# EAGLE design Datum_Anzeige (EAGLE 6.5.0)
dasdad
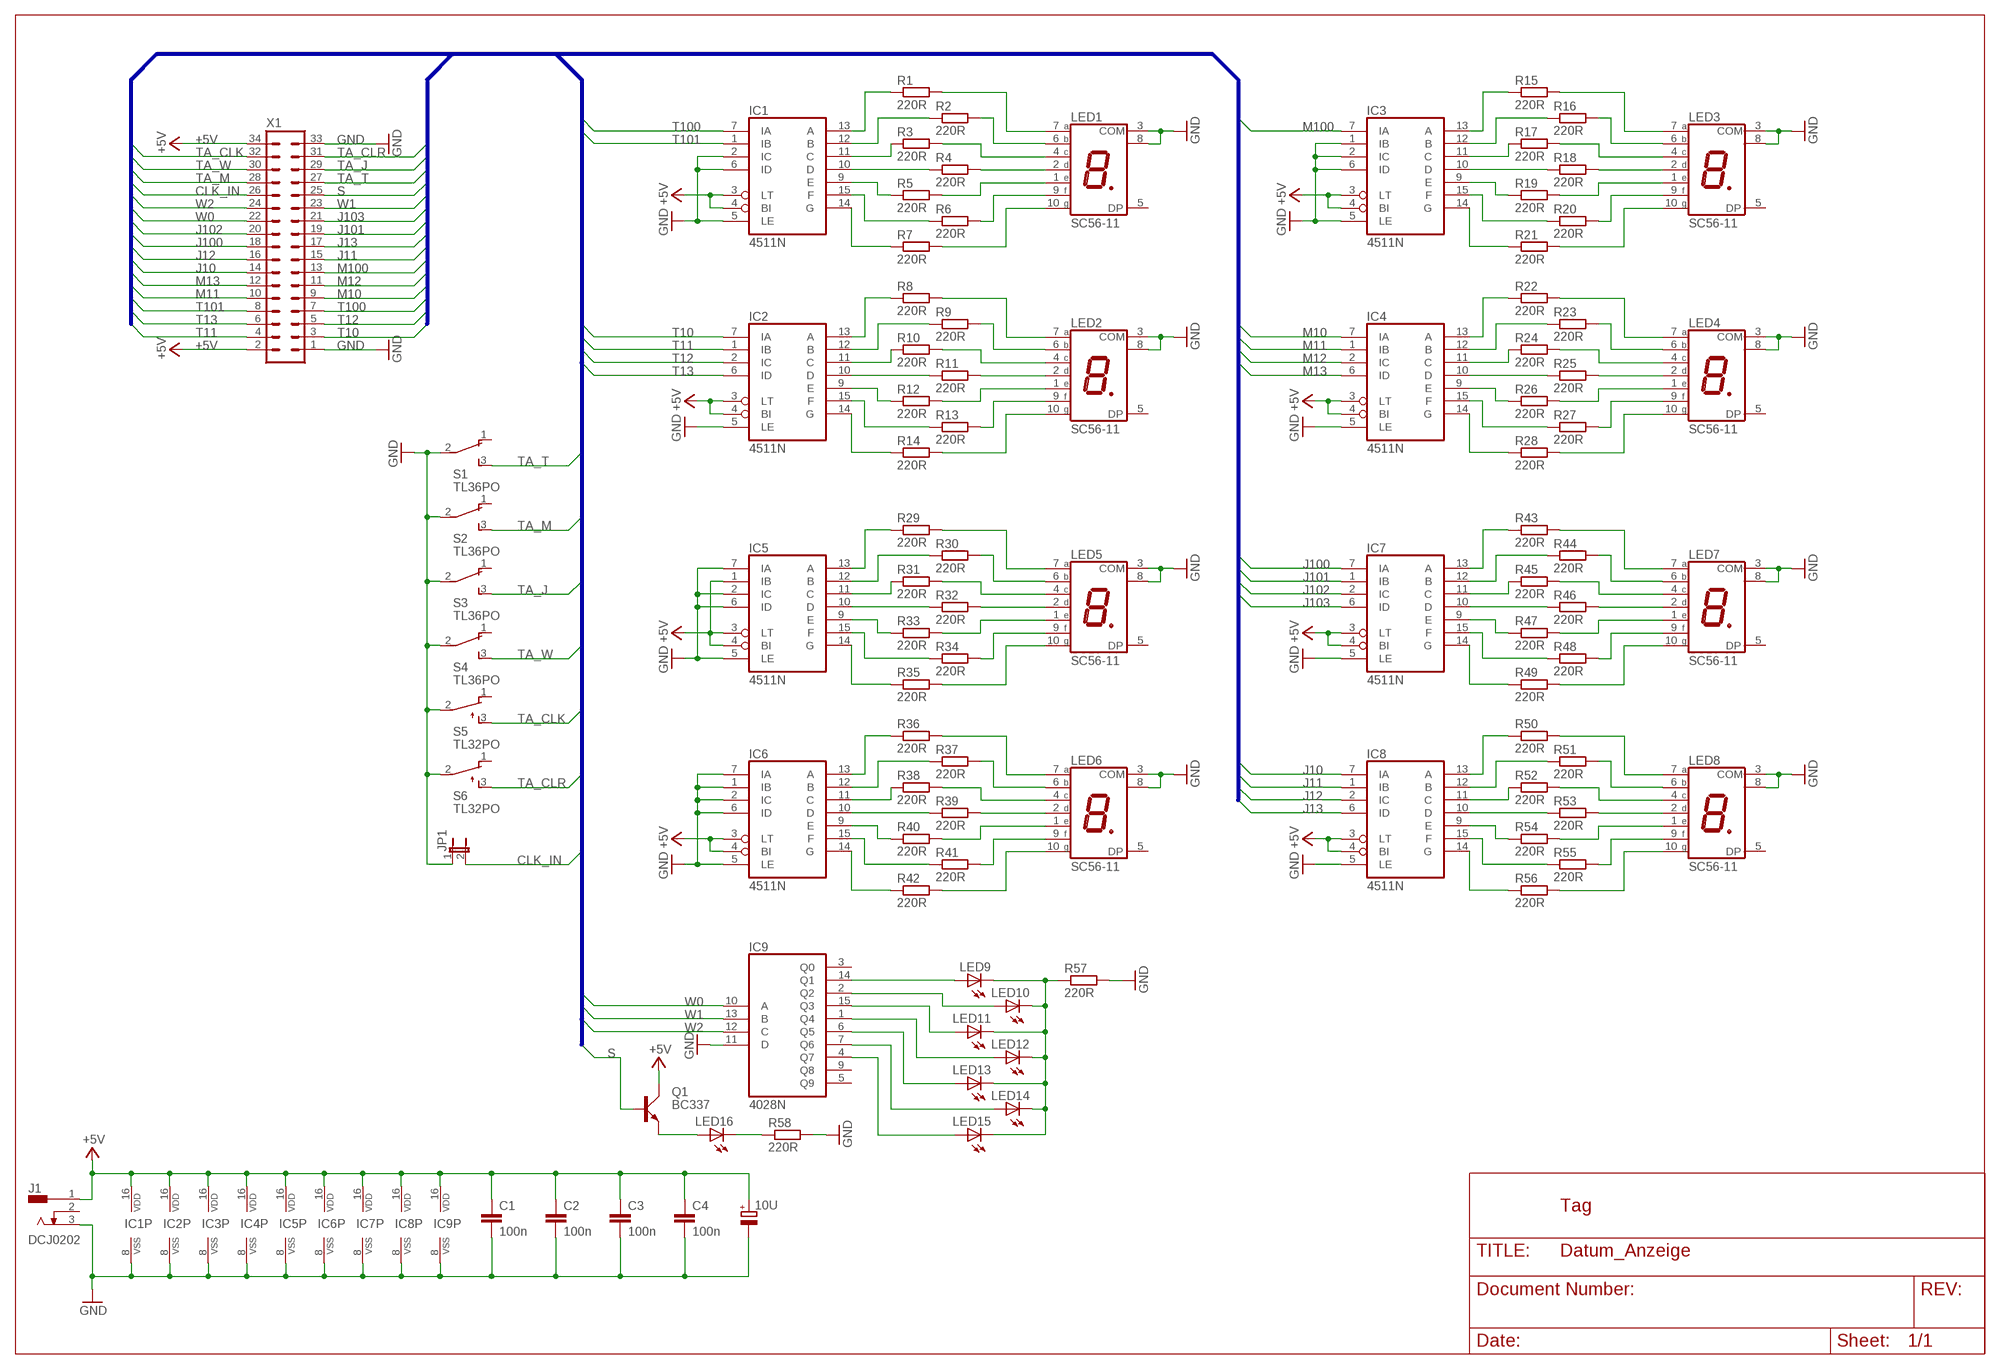
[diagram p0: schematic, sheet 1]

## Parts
10U  CPOL-EUE2.5-7  [E2,5-7]
C1  100n  C-EU025-024X044  [C025-024X044]
C2  100n  C-EU025-024X044  [C025-024X044]
C3  100n  C-EU025-024X044  [C025-024X044]
C4  100n  C-EU025-024X044  [C025-024X044]
IC1  4511N  [DIL16]
IC2  4511N  [DIL16]
IC3  4511N  [DIL16]
IC4  4511N  [DIL16]
IC5  4511N  [DIL16]
IC6  4511N  [DIL16]
IC7  4511N  [DIL16]
IC8  4511N  [DIL16]
IC9  4028N  [DIL16]
J1  DCJ0202  [DCJ0202]
JP1  JP1E  [JP1]
LED1  SC56-11  7-SEG_SA56-11  [SA56-11]
LED2  SC56-11  7-SEG_SA56-11  [SA56-11]
LED3  SC56-11  7-SEG_SA56-11  [SA56-11]
LED4  SC56-11  7-SEG_SA56-11  [SA56-11]
LED5  SC56-11  7-SEG_SA56-11  [SA56-11]
LED6  SC56-11  7-SEG_SA56-11  [SA56-11]
LED7  SC56-11  7-SEG_SA56-11  [SA56-11]
LED8  SC56-11  7-SEG_SA56-11  [SA56-11]
LED9  LED5MM  [LED5MM]
LED10  LED5MM  [LED5MM]
LED11  LED5MM  [LED5MM]
LED12  LED5MM  [LED5MM]
LED13  LED5MM  [LED5MM]
LED14  LED5MM  [LED5MM]
LED15  LED5MM  [LED5MM]
LED16  LED5MM  [LED5MM]
Q1  BC337  [SOT54A]
R1  220R  R-EU_0204/5  [0204/5]
R2  220R  R-EU_0204/5  [0204/5]
R3  220R  R-EU_0204/5  [0204/5]
R4  220R  R-EU_0204/5  [0204/5]
R5  220R  R-EU_0204/5  [0204/5]
R6  220R  R-EU_0204/5  [0204/5]
R7  220R  R-EU_0204/5  [0204/5]
R8  220R  R-EU_0204/5  [0204/5]
R9  220R  R-EU_0204/5  [0204/5]
R10  220R  R-EU_0204/5  [0204/5]
R11  220R  R-EU_0204/5  [0204/5]
R12  220R  R-EU_0204/5  [0204/5]
R13  220R  R-EU_0204/5  [0204/5]
R14  220R  R-EU_0204/5  [0204/5]
R15  220R  R-EU_0204/5  [0204/5]
R16  220R  R-EU_0204/5  [0204/5]
R17  220R  R-EU_0204/5  [0204/5]
R18  220R  R-EU_0204/5  [0204/5]
R19  220R  R-EU_0204/5  [0204/5]
R20  220R  R-EU_0204/5  [0204/5]
R21  220R  R-EU_0204/5  [0204/5]
R22  220R  R-EU_0204/5  [0204/5]
R23  220R  R-EU_0204/5  [0204/5]
R24  220R  R-EU_0204/5  [0204/5]
R25  220R  R-EU_0204/5  [0204/5]
R26  220R  R-EU_0204/5  [0204/5]
R27  220R  R-EU_0204/5  [0204/5]
R28  220R  R-EU_0204/5  [0204/5]
R29  220R  R-EU_0204/5  [0204/5]
R30  220R  R-EU_0204/5  [0204/5]
R31  220R  R-EU_0204/5  [0204/5]
R32  220R  R-EU_0204/5  [0204/5]
R33  220R  R-EU_0204/5  [0204/5]
R34  220R  R-EU_0204/5  [0204/5]
R35  220R  R-EU_0204/5  [0204/5]
R36  220R  R-EU_0204/5  [0204/5]
R37  220R  R-EU_0204/5  [0204/5]
R38  220R  R-EU_0204/5  [0204/5]
R39  220R  R-EU_0204/5  [0204/5]
R40  220R  R-EU_0204/5  [0204/5]
R41  220R  R-EU_0204/5  [0204/5]
R42  220R  R-EU_0204/5  [0204/5]
R43  220R  R-EU_0204/5  [0204/5]
R44  220R  R-EU_0204/5  [0204/5]
R45  220R  R-EU_0204/5  [0204/5]
R46  220R  R-EU_0204/5  [0204/5]
R47  220R  R-EU_0204/5  [0204/5]
R48  220R  R-EU_0204/5  [0204/5]
R49  220R  R-EU_0204/5  [0204/5]
R50  220R  R-EU_0204/5  [0204/5]
R51  220R  R-EU_0204/5  [0204/5]
R52  220R  R-EU_0204/5  [0204/5]
R53  220R  R-EU_0204/5  [0204/5]
R54  220R  R-EU_0204/5  [0204/5]
R55  220R  R-EU_0204/5  [0204/5]
R56  220R  R-EU_0204/5  [0204/5]
R57  220R  R-EU_0204/5  [0204/5]
R58  220R  R-EU_0204/5  [0204/5]
S1  TL36PO  [TL3XPO]
S2  TL36PO  [TL3XPO]
S3  TL36PO  [TL3XPO]
S4  TL36PO  [TL3XPO]
S5  TL32PO  [TL3XPO]
S6  TL32PO  [TL3XPO]
X1  ML34  [ML34]

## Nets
+5V: 10U.+ C1.1 C2.1 C3.1 C4.1 IC1.3(LT) IC1.4(BI) IC1.16(VDD) IC2.3(LT) IC2.4(BI) IC2.16(VDD) IC3.3(LT) IC3.4(BI) IC3.16(VDD) IC4.3(LT) IC4.4(BI) IC4.16(VDD) IC5.1(IB) IC5.3(LT) IC5.4(BI) IC5.16(VDD) IC6.3(LT) IC6.4(BI) IC6.16(VDD) IC7.3(LT) IC7.4(BI) IC7.16(VDD) IC8.3(LT) IC8.4(BI) IC8.16(VDD) IC9.16(VDD) J1.1 Q1.C X1.2 X1.34
CLK_IN: JP1.2 X1.26
GND: 10U.- C1.2 C2.2 C3.2 C4.2 IC1.2(IC) IC1.5(LE) IC1.6(ID) IC1.8(VSS) IC2.5(LE) IC2.8(VSS) IC3.1(IB) IC3.2(IC) IC3.5(LE) IC3.6(ID) IC3.8(VSS) IC4.5(LE) IC4.8(VSS) IC5.2(IC) IC5.5(LE) IC5.6(ID) IC5.7(IA) IC5.8(VSS) IC6.1(IB) IC6.2(IC) IC6.5(LE) IC6.6(ID) IC6.7(IA) IC6.8(VSS) IC7.5(LE) IC7.8(VSS) IC8.5(LE) IC8.8(VSS) IC9.8(VSS) IC9.11(D) J1.3 JP1.1 LED1.3(COM) LED1.8(COM) LED2.3(COM) LED2.8(COM) LED3.3(COM) LED3.8(COM) LED4.3(COM) LED4.8(COM) LED5.3(COM) LED5.8(COM) LED6.3(COM) LED6.8(COM) LED7.3(COM) LED7.8(COM) LED8.3(COM) LED8.8(COM) R57.2 R58.2 S1.2(P) S2.2(P) S3.2(P) S4.2(P) S5.2(P) S6.2(P) X1.1 X1.33
J10: IC8.7(IA) X1.14
J11: IC8.1(IB) X1.15
J12: IC8.2(IC) X1.16
J13: IC8.6(ID) X1.17
J100: IC7.7(IA) X1.18
J101: IC7.1(IB) X1.19
J102: IC7.2(IC) X1.20
J103: IC7.6(ID) X1.21
M10: IC4.7(IA) X1.9
M11: IC4.1(IB) X1.10
M12: IC4.2(IC) X1.11
M13: IC4.6(ID) X1.12
M100: IC3.7(IA) X1.13
N$1: IC1.13(A) R1.1
N$2: LED9.K(C) LED10.K(C) LED11.K(C) LED12.K(C) LED13.K(C) LED14.K(C) LED15.K(C) R57.1
N$3: IC1.12(B) R2.1
N$4: IC1.11(C) R3.1
N$5: IC1.10(D) R4.1
N$6: IC1.9(E) R5.1
N$7: IC1.15(F) R6.1
N$8: IC1.14(G) R7.1
N$9: LED1.2(D) R4.2
N$10: LED1.4(C) R3.2
N$11: LED1.6(B) R2.2
N$12: IC9.2(Q2) LED10.A
N$13: LED1.7(A) R1.2
N$14: LED1.1(E) R5.2
N$15: LED1.9(F) R6.2
N$16: LED1.10(G) R7.2
N$17: IC2.13(A) R8.1
N$18: IC2.12(B) R9.1
N$19: IC2.11(C) R10.1
N$20: IC2.10(D) R11.1
N$21: IC2.9(E) R12.1
N$22: IC2.15(F) R13.1
N$23: IC2.14(G) R14.1
N$24: LED2.2(D) R11.2
N$25: LED2.4(C) R10.2
N$26: LED2.6(B) R9.2
N$27: LED2.7(A) R8.2
N$28: LED2.1(E) R12.2
N$29: LED2.9(F) R13.2
N$30: LED2.10(G) R14.2
N$31: IC9.14(Q1) LED9.A
N$32: IC3.13(A) R15.1
N$33: IC3.12(B) R16.1
N$34: IC3.11(C) R17.1
N$35: IC3.10(D) R18.1
N$36: IC3.9(E) R19.1
N$37: IC3.15(F) R20.1
N$38: IC3.14(G) R21.1
N$39: LED3.2(D) R18.2
N$40: LED3.4(C) R17.2
N$41: LED3.6(B) R16.2
N$42: LED3.7(A) R15.2
N$43: LED3.1(E) R19.2
N$44: LED3.9(F) R20.2
N$45: LED3.10(G) R21.2
N$46: IC4.13(A) R22.1
N$47: IC4.12(B) R23.1
N$48: IC4.11(C) R24.1
N$49: IC4.10(D) R25.1
N$50: IC4.9(E) R26.1
N$51: IC4.15(F) R27.1
N$52: IC4.14(G) R28.1
N$53: LED4.2(D) R25.2
N$54: LED4.4(C) R24.2
N$55: LED4.6(B) R23.2
N$56: LED4.7(A) R22.2
N$57: LED4.1(E) R26.2
N$58: LED4.9(F) R27.2
N$59: LED4.10(G) R28.2
N$60: IC5.13(A) R29.1
N$61: IC5.12(B) R30.1
N$62: IC5.11(C) R31.1
N$63: IC5.10(D) R32.1
N$64: IC5.9(E) R33.1
N$65: IC5.15(F) R34.1
N$66: IC5.14(G) R35.1
N$67: LED5.2(D) R32.2
N$68: LED5.4(C) R31.2
N$69: LED5.6(B) R30.2
N$70: LED5.7(A) R29.2
N$71: LED5.1(E) R33.2
N$72: LED5.9(F) R34.2
N$73: LED5.10(G) R35.2
N$74: IC6.13(A) R36.1
N$75: IC6.12(B) R37.1
N$76: IC6.11(C) R38.1
N$77: IC6.10(D) R39.1
N$78: IC6.9(E) R40.1
N$79: IC6.15(F) R41.1
N$80: IC6.14(G) R42.1
N$81: LED6.2(D) R39.2
N$82: LED6.4(C) R38.2
N$83: LED6.6(B) R37.2
N$84: LED6.7(A) R36.2
N$85: LED6.1(E) R40.2
N$86: LED6.9(F) R41.2
N$87: LED6.10(G) R42.2
N$88: IC7.13(A) R43.1
N$89: IC7.12(B) R44.1
N$90: IC7.11(C) R45.1
N$91: IC7.10(D) R46.1
N$92: IC7.9(E) R47.1
N$93: IC7.15(F) R48.1
N$94: IC7.14(G) R49.1
N$95: LED7.2(D) R46.2
N$96: LED7.4(C) R45.2
N$97: LED7.6(B) R44.2
N$98: LED7.7(A) R43.2
N$99: LED7.1(E) R47.2
N$100: LED7.9(F) R48.2
N$101: LED7.10(G) R49.2
N$102: IC8.13(A) R50.1
N$103: IC8.12(B) R51.1
N$104: IC8.11(C) R52.1
N$105: IC8.10(D) R53.1
N$106: IC8.9(E) R54.1
N$107: IC8.15(F) R55.1
N$108: IC8.14(G) R56.1
N$109: LED8.2(D) R53.2
N$110: LED8.4(C) R52.2
N$111: LED8.6(B) R51.2
N$112: LED8.7(A) R50.2
N$113: LED8.1(E) R54.2
N$114: LED8.9(F) R55.2
N$115: LED8.10(G) R56.2
N$116: IC9.15(Q3) LED11.A
N$117: IC9.1(Q4) LED12.A
N$118: IC9.6(Q5) LED13.A
N$119: IC9.7(Q6) LED14.A
N$120: IC9.4(Q7) LED15.A
N$121: LED16.K(C) R58.1
N$123: LED16.A Q1.E
S: Q1.B X1.25
T10: IC2.7(IA) X1.3
T11: IC2.1(IB) X1.4
T12: IC2.2(IC) X1.5
T13: IC2.6(ID) X1.6
T100: IC1.7(IA) X1.7
T101: IC1.1(IB) X1.8
TA_CLK: S5.3(S) X1.32
TA_CLR: S6.3(S) X1.31
TA_J: S3.3(S) X1.29
TA_M: S2.3(S) X1.28
TA_T: S1.3(S) X1.27
TA_W: S4.3(S) X1.30
W0: IC9.10(A) X1.22
W1: IC9.13(B) X1.23
W2: IC9.12(C) X1.24
Unconnected: IC9.3(Q0) IC9.5(Q9) IC9.9(Q8) J1.2 LED1.5(DP) LED2.5(DP) LED3.5(DP) LED4.5(DP) LED5.5(DP) LED6.5(DP) LED7.5(DP) LED8.5(DP) S1.1(O) S2.1(O) S3.1(O) S4.1(O) S5.1(O) S6.1(O)

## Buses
T10,T11,T12,T13,T100,T101,M100,M10,M11,M12,M13,J100,J101,J102,J103,J10,J11,J12,J13,W0,W1,W2,S,CLK_IN,TA_T,TA_M,TA_J,TA_W,TA_CLK,TA_CLR

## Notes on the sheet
- Tag

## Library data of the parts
10U = rcl:CPOL-EU: POLARIZED CAPACITOR, European symbol
C1-C4 = rcl:C-EU: CAPACITOR, European symbol
IC1-IC8 = 45xx:4511: BCD to 7-segment LATCH/DECODER/DRIVER
IC9 = 40xx:4028: BCD to decimal DECODER
J1 = Brunner:DCJ0202: DC POWER JACK Source: DCJ0202.pdf; OC_FARNELL: unknown; OC_NEWARK: unknown
JP1 = jumper:JP1E: JUMPER
LED1-LED8 = display-kingbright:7-SEG_: Kingbright 14.2mm (0.56 INCH) SINGLE DIGIT NUMERIC DUISPLAY Source: SA56-11EWA(Ver1189471036.pdf; OC_FARNELL: unknown; OC_NEWARK: unknown
LED9-LED16 = led:LED: LED
Q1 = transistor-small-signal:BC337: NPN TRANSISTOR
R1-R58 = rcl:R-EU_: RESISTOR, European symbol
S1-S4 = switch:TL36PO: TINY SWITCH ON - ON Source: http://www2.produktinfo.conrad.com/datenblaetter/700000-724999/705152-da-01-de-Subminiaturschalter_TL_36YO.pdf
S5 S6 = switch:TL32PO: TINY SWITCH ON - MOM Source: http://www2.produktinfo.conrad.com/datenblaetter/700000-724999/705152-da-01-de-Subminiaturschalter_TL_36YO.pdf
X1 = con-harting-ml:ML34: HARTING; OC_FARNELL: unknown; OC_NEWARK: unknown

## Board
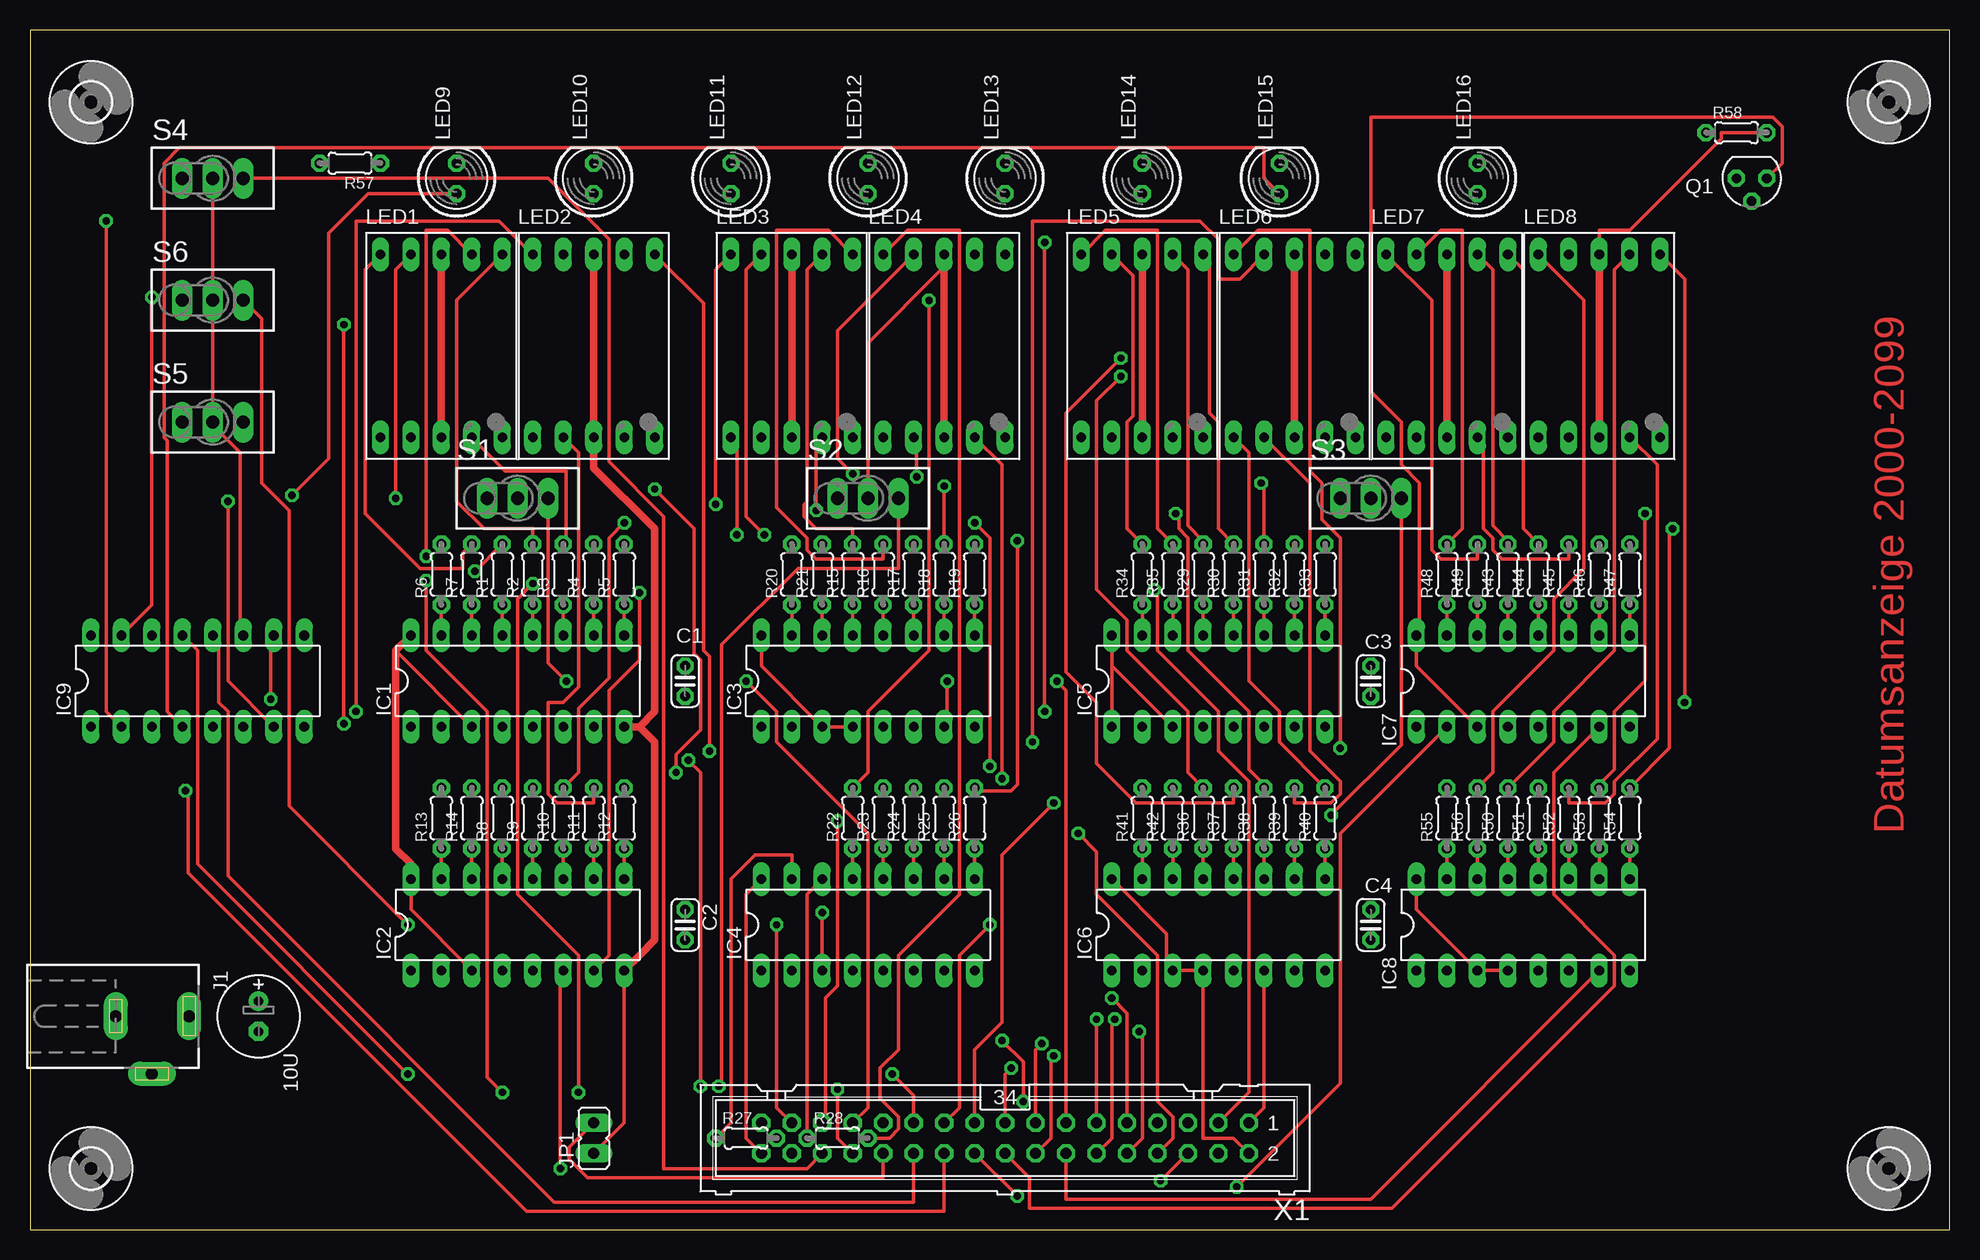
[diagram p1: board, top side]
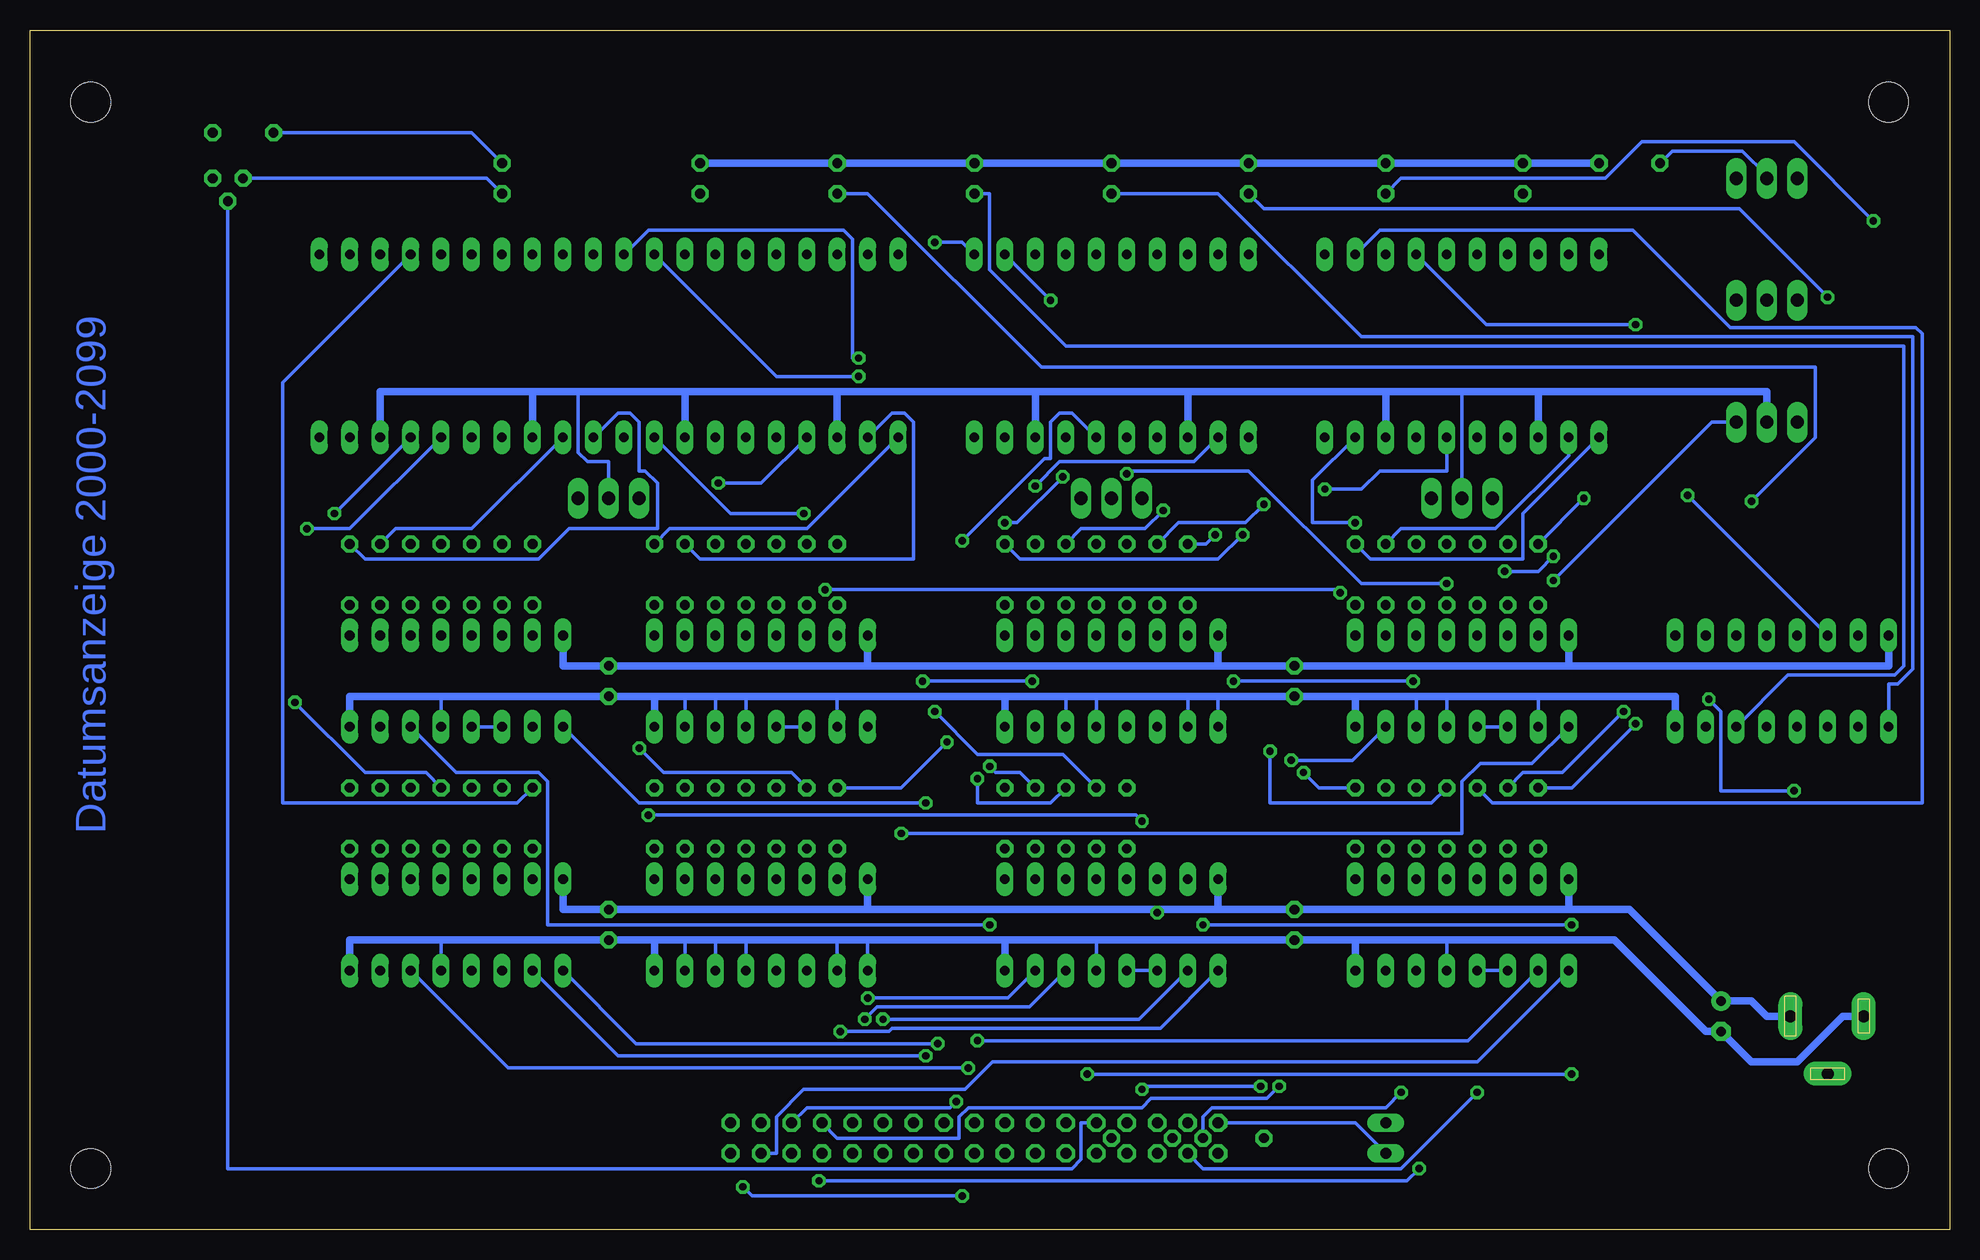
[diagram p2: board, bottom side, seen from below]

Size 160 x 100 mm. Coordinates in mm from the lower left corner, seen from the top.
Outline: 0,0 160,0 160,100 0,100 0,0
Copper layers (1*16): Top 0.035mm / dielectric 1.5mm / Bottom 0.035mm
Design rules "default *": minimum track width 12mil, minimum drill 24mil, track to track 12mil, track to pad 12mil, pad to pad 12mil, via to via 12mil, smd to smd 8mil, copper to edge 40mil, drill to drill 8mil, minimum pad ring 12mil, minimum via ring 10mil, stop-mask expansion 4mil, vias tented up to drill 0mil, thermal gap 10mil

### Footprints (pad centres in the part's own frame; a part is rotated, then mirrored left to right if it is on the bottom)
E2,5-7 = drill 0.813 pad 1.6: + -1.27,0 | drill 0.813 pad 1.6 octagon: - 1.27,0
C025-024X044 = drill 0.813 octagon: 1 -1.27,0; 2 1.27,0
DIL16 = drill 0.813 long: 1 -8.89,-3.81; 2 -6.35,-3.81; 3 -3.81,-3.81; 4 -1.27,-3.81; 5 1.27,-3.81; 6 3.81,-3.81; 7 6.35,-3.81; 8 8.89,-3.81; 9 8.89,3.81; 10 6.35,3.81; 11 3.81,3.81; 12 1.27,3.81; 13 -1.27,3.81; 14 -3.81,3.81; 15 -6.35,3.81; 16 -8.89,3.81
DCJ0202 = drill 1 pad 2 long: 1 0,3.1; 2 4.8,0; 3 0,-3
JP1 = drill 0.914 long: 1 0,-1.27; 2 0,1.27
SA56-11 = drill 0.8 long: 1 -5.08,-7.62; 2 -2.54,-7.62; 3 0,-7.62; 4 2.54,-7.62; 5 5.08,-7.62; 6 5.08,7.62; 7 2.54,7.62; 8 0,7.62; 9 -2.54,7.62; 10 -5.08,7.62
LED5MM = drill 0.813 octagon: A -1.27,0; K 1.27,0
SOT54A = drill 0.813 octagon: B 0,1.905; C -1.27,0; E 1.27,0
0204/5 = drill 0.813 octagon: 1 -2.54,0; 2 2.54,0
TL3XPO = drill 1.1 pad 1.422 long: 1 -2.54,0; 2 0,0; 3 2.54,0
3,3 = hole 3.3: 0,0
ML34 = drill 0.914 octagon: 1 -20.32,-1.27; 2 -20.32,1.27; 3 -17.78,-1.27; 4 -17.78,1.27; 5 -15.24,-1.27; 6 -15.24,1.27; 7 -12.7,-1.27; 8 -12.7,1.27; 9 -10.16,-1.27; 10 -10.16,1.27; 11 -7.62,-1.27; 12 -7.62,1.27; 13 -5.08,-1.27; 14 -5.08,1.27; 15 -2.54,-1.27; 16 -2.54,1.27; 17 0,-1.27; 18 0,1.27; 19 2.54,-1.27; 20 2.54,1.27; 21 5.08,-1.27; 22 5.08,1.27; 23 7.62,-1.27; 24 7.62,1.27; 25 10.16,-1.27; 26 10.16,1.27; 27 12.7,-1.27; 28 12.7,1.27; 29 15.24,-1.27; 30 15.24,1.27; 31 17.78,-1.27; 32 17.78,1.27; 33 20.32,-1.27; 34 20.32,1.27

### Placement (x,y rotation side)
10U  19.05,17.78 270 top
C1  54.61,45.72 270 top
C2  54.61,25.4 270 top
C3  111.76,45.72 270 top
C4  111.76,25.4 270 top
IC1  40.64,45.72 0 top
IC2  40.64,25.4 0 top
IC3  69.85,45.72 0 top
IC4  69.85,25.4 0 top
IC5  99.06,45.72 0 top
IC6  99.06,25.4 0 top
IC7  124.46,45.72 0 top
IC8  124.46,25.4 0 top
IC9  13.97,45.72 0 top
J1  10.16,17.78 270 top
JP1  46.99,7.62 0 top
LED1  34.29,73.66 0 top
LED2  46.99,73.66 0 top
LED3  63.5,73.66 0 top
LED4  76.2,73.66 0 top
LED5  92.71,73.66 0 top
LED6  105.41,73.66 0 top
LED7  118.11,73.66 0 top
LED8  130.81,73.66 0 top
LED9  35.56,87.63 90 top
LED10  46.99,87.63 90 top
LED11  58.42,87.63 90 top
LED12  69.85,87.63 90 top
LED13  81.28,87.63 90 top
LED14  92.71,87.63 90 top
LED15  104.14,87.63 90 top
LED16  120.65,87.63 90 top
Q1  143.51,87.63 180 top
R1  39.37,54.61 90 top
R2  41.91,54.61 90 top
R3  44.45,54.61 90 top
R4  46.99,54.61 90 top
R5  49.53,54.61 90 top
R6  34.29,54.61 90 top
R7  36.83,54.61 90 top
R8  39.37,34.29 90 top
R9  41.91,34.29 90 top
R10  44.45,34.29 90 top
R11  46.99,34.29 90 top
R12  49.53,34.29 90 top
R13  34.29,34.29 90 top
R14  36.83,34.29 90 top
R15  68.58,54.61 90 top
R16  71.12,54.61 90 top
R17  73.66,54.61 90 top
R18  76.2,54.61 90 top
R19  78.74,54.61 90 top
R20  63.5,54.61 90 top
R21  66.04,54.61 90 top
R22  68.58,34.29 90 top
R23  71.12,34.29 90 top
R24  73.66,34.29 90 top
R25  76.2,34.29 90 top
R26  78.74,34.29 90 top
R27  59.69,7.62 0 top
R28  67.31,7.62 0 top
R29  97.79,54.61 90 top
R30  100.33,54.61 90 top
R31  102.87,54.61 90 top
R32  105.41,54.61 90 top
R33  107.95,54.61 90 top
R34  92.71,54.61 90 top
R35  95.25,54.61 90 top
R36  97.79,34.29 90 top
R37  100.33,34.29 90 top
R38  102.87,34.29 90 top
R39  105.41,34.29 90 top
R40  107.95,34.29 90 top
R41  92.71,34.29 90 top
R42  95.25,34.29 90 top
R43  123.19,54.61 90 top
R44  125.73,54.61 90 top
R45  128.27,54.61 90 top
R46  130.81,54.61 90 top
R47  133.35,54.61 90 top
R48  118.11,54.61 90 top
R49  120.65,54.61 90 top
R50  123.19,34.29 90 top
R51  125.73,34.29 90 top
R52  128.27,34.29 90 top
R53  130.81,34.29 90 top
R54  133.35,34.29 90 top
R55  118.11,34.29 90 top
R56  120.65,34.29 90 top
R57  26.67,88.9 180 top
R58  142.24,91.44 0 top
S1  40.64,60.96 0 top
S2  69.85,60.96 0 top
S3  111.76,60.96 0 top
S4  15.24,87.63 0 top
S5  15.24,67.31 0 top
S6  15.24,77.47 0 top
U$1  [3,3]  5.08,93.98 0 top
U$2  [3,3]  5.08,5.08 0 top
U$3  [3,3]  154.94,93.98 0 top
U$4  [3,3]  154.94,5.08 0 top
U$5  [A4L-LOC]  not placed on the board
X1  81.28,7.62 180 top

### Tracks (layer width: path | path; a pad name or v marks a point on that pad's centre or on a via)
+5V  (via drill 0.61)
  Top 0.305: X1.2 100.33,7.62 97.79,7.62 IC6.4 IC6.3 94.74,22.1 94.74,24.64 IC6.16 | IC8.4 IC8.3 115.57,26.67 IC8.16 | IC3.4 IC3.3 60.96,46.99 IC3.16 | IC5.16 90.17,46.99 | 90.17,46.99 IC5.1 | Q1.C 146.05,88.9 146.05,91.95 145.29,92.71 111.76,92.71 111.76,69.85 114.3,67.31 114.3,63.75 115.82,62.23 115.82,49.78 IC7.16 115.57,46.99 IC7.3 | X1.34 59.69,7.62 59.69,27.94 IC4.16 | IC2.3 31.75,26.67 31.75,28.96 IC2.16 | IC1.3 30.73,48.01 30.48,48.01 | v66.04,26.42 IC4.3 | 90.17,46.99 IC5.3
  Top 0.61: IC2.16 31.75,30.48 30.48,31.75 30.48,48.01 30.48,48.26 IC1.16
  Bottom 0.305: IC7.4 IC7.3 | IC5.4 IC5.3 | IC4.4 IC4.3 | IC1.4 IC1.3 | IC2.4 IC2.3 | v66.04,26.42 66.04,26.67
  Bottom 0.61: IC9.16 5.08,46.99 31.75,46.99 | 31.75,46.99 C1.1 60.96,46.99 | 60.96,46.99 90.17,46.99 | 90.17,46.99 C3.1 115.57,46.99 IC7.16 | IC5.16 90.17,46.99 | IC3.16 60.96,48.26 60.96,46.99 | IC1.16 31.75,46.99 | IC2.16 31.75,26.67 | 31.75,26.67 C2.1 60.96,26.67 | 60.96,26.67 66.04,26.67 90.17,26.67 | 90.17,26.67 C4.1 115.57,26.67 IC8.16 | IC6.16 90.17,26.67 | IC4.16 60.96,26.67 | 31.75,26.67 26.67,26.67 10U.+ 16.51,19.05 15.24,17.78 J1.1
CLK_IN
  Top 0.305: JP1.2 44.96,6.86 44.96,5.84 46.48,4.32 71.12,4.32 X1.26
GND
  Top 0.305: S4.2 S6.2 S5.2 15.24,67.06 17.53,64.77 17.53,49.78 IC9.11 | R58.2 140.97,91.44 140.97,90.93 133.35,83.31 130.81,83.31 130.81,81.53 LED8.8 | X1.1 102.87,10.16 IC6.6 | S2.2 69.85,73.91 75.95,80.01 LED4.8 | JP1.1 49.53,8.89 49.53,21.34 IC2.8
  Top 0.61: IC2.8 50.8,22.86 52.07,24.13 52.07,40.64 50.8,41.91 | 50.8,41.91 IC1.8 50.8,41.91 | LED1.8 LED1.3 | LED2.8 LED2.3 46.99,63.5 52.07,58.42 52.07,43.18 50.8,41.91 | LED3.8 LED3.3 | LED4.8 LED4.3 | LED5.8 LED5.3 | LED6.8 LED6.3 | LED7.8 LED7.3 | LED8.8 LED8.3
  Bottom 0.305: R57.2 23.11,89.92 17.27,89.92 15.24,87.88 S4.2 | JP1.1 49.53,8.89 X1.33 | IC2.5 41.91,23.88 41.91,24.13 | IC1.2 34.29,44.2 34.29,44.45 | IC1.5 41.91,44.2 41.91,44.45 | IC1.6 44.45,44.2 44.45,44.45 | IC4.5 71.12,23.88 71.12,24.13 | IC3.1 60.96,44.2 60.96,44.45 | IC3.2 63.5,44.2 63.5,44.45 | IC3.5 71.12,44.2 71.12,44.45 | IC3.6 73.66,44.2 73.66,44.45 | IC6.1 90.17,23.88 90.17,24.13 | IC6.2 92.71,23.88 92.71,24.13 | IC5.2 92.71,44.2 92.71,44.45 | IC6.5 100.33,23.88 100.33,24.13 | IC6.6 102.87,23.88 102.87,24.13 | IC6.7 105.41,23.88 105.41,24.13 | IC8.5 125.73,23.88 125.73,24.13 | IC5.5 100.33,44.2 100.33,44.45 | IC5.6 102.87,44.2 102.87,44.45 | IC5.7 105.41,44.2 105.41,44.45 | IC7.5 125.73,44.2 125.73,44.45 | S1.2 40.64,69.6 40.64,69.85 | S3.2 111.76,64.01 113.54,64.01 114.3,64.77 114.3,69.6 114.3,69.85
  Bottom 0.61: IC9.8 22.86,44.45 34.29,44.45 41.91,44.45 44.45,44.45 49.53,44.45 | 49.53,44.45 C1.2 60.96,44.45 63.5,44.45 71.12,44.45 73.66,44.45 78.74,44.45 | 78.74,44.45 92.71,44.45 100.33,44.45 102.87,44.45 105.41,44.45 107.95,44.45 | 107.95,44.45 C3.2 125.73,44.45 133.35,44.45 IC7.8 | IC5.8 107.95,44.45 | IC3.8 78.74,44.45 | IC1.8 49.53,44.45 | IC2.8 49.53,24.13 | 49.53,24.13 C2.2 71.12,24.13 78.74,24.13 | 78.74,24.13 90.17,24.13 92.71,24.13 100.33,24.13 102.87,24.13 105.41,24.13 107.95,24.13 | 107.95,24.13 C4.2 125.73,24.13 133.35,24.13 IC8.8 | IC6.8 107.95,24.13 | IC4.8 78.74,24.13 | 49.53,24.13 41.91,24.13 27.94,24.13 20.32,16.51 10U.- 17.78,15.24 16.51,13.97 12.7,13.97 8.89,17.78 7.62,17.78 J1.3 | S5.2 15.24,69.85 34.29,69.85 | 34.29,69.85 40.64,69.85 46.99,69.85 | 46.99,69.85 63.5,69.85 | 63.5,69.85 76.2,69.85 | 76.2,69.85 92.71,69.85 | 92.71,69.85 105.41,69.85 | 105.41,69.85 114.3,69.85 118.11,69.85 | 118.11,69.85 130.81,69.85 LED8.3 | LED7.3 118.11,69.85 | LED6.3 105.41,69.85 | LED5.3 92.71,69.85 | LED4.3 76.2,69.85 | LED3.3 63.5,69.85 | LED2.3 46.99,69.85 | LED1.3 34.29,69.85
J10
  Top 0.305: IC8.7 111.76,2.54 86.36,2.54 X1.14
J11  (via drill 0.61)
  Top 0.305: v84.33,15.49 83.82,14.99 X1.15
  Bottom 0.305: IC8.1 109.47,15.49 v84.33,15.49
J12  (via drill 0.61)
  Top 0.305: v85.34,14.48 85.09,14.22 85.09,7.62 X1.16
  Bottom 0.305: IC8.2 111,14.48 v85.34,14.48
J13  (via drill 0.61)
  Top 0.305: v81.79,13.46 81.28,12.95 X1.17
  Bottom 0.305: IC8.6 120.14,13.46 v81.79,13.46
J100
  Top 0.305: IC7.7 127,38.1 127,27.94 132.08,22.86 132.08,20.32 113.54,1.78 83.31,1.78 83.31,4.32 X1.18
J101  (via drill 0.61)
  Top 0.305: v85.34,35.56 81.03,31.24 81.03,17.27 78.74,14.99 X1.19
  Bottom 0.305: IC7.1 109.22,35.56 v85.34,35.56
J102  (via drill 0.61)
  Top 0.305: IC7.2 109.22,33.02 109.22,12.19 v100.58,3.56 | X1.20 v82.3,2.79
  Bottom 0.305: v100.58,3.56 99.82,2.79 v82.3,2.79
J103  (via drill 0.61)
  Top 0.305: v80.01,25.4 77.47,22.86 77.47,10.16 X1.21
  Bottom 0.305: IC7.6 124.46,38.1 117.6,38.1 116.84,37.34 116.84,25.4 v80.01,25.4
M10  (via drill 0.61)
  Top 0.305: v90.17,19.3 91.44,18.03 X1.9
  Bottom 0.305: IC4.7 78.49,19.3 v90.17,19.3
M11  (via drill 0.61)
  Top 0.305: v92.46,16.51 92.71,16.26 92.71,7.62 X1.10
  Bottom 0.305: IC4.1 65.79,16.76 88.14,16.76 88.39,16.51 v92.46,16.51
M12  (via drill 0.61)
  Top 0.305: X1.11 v88.9,17.53
  Bottom 0.305: IC4.2 67.56,17.53 v88.9,17.53
M13  (via drill 0.61)
  Top 0.305: v90.42,17.53 90.17,17.27 90.17,7.62 X1.12
  Bottom 0.305: IC4.6 76.71,18.54 89.41,18.54 v90.42,17.53
M100  (via drill 0.61)
  Top 0.305: IC3.7 76.45,42.16 v76.45,45.72 | v85.6,45.72 86.36,44.96 X1.13
  Bottom 0.305: v85.6,45.72 v76.45,45.72
N$1
  Top 0.305: R1.1 IC1.13
N$2
  Bottom 0.61: LED15.K LED14.K LED13.K LED12.K LED11.K LED10.K LED9.K R57.1
N$3
  Top 0.305: R2.1 IC1.12
N$4
  Top 0.305: R3.1 IC1.11
N$5
  Top 0.305: R4.1 IC1.10
N$6
  Top 0.305: R5.1 IC1.9
N$7
  Top 0.305: R6.1 IC1.15
N$8
  Top 0.305: R7.1 IC1.14
N$9
  Bottom 0.305: LED1.2 31.75,64.52 37.85,58.42 45.72,58.42 R4.2
N$10
  Top 0.305: LED1.4 39.62,63.25 44.7,63.25 44.7,57.4 R3.2
N$11
  Top 0.305: LED1.6 35.56,77.47 35.56,60.71 37.85,58.42 41.91,58.42 R2.2
N$12  (via drill 0.61)
  Top 0.305: IC9.2 6.35,43.18 v6.35,84.07
  Bottom 0.305: v6.35,84.07 12.95,90.68 25.65,90.68 28.7,87.63 45.72,87.63 LED10.A
N$13  (via drill 0.61)
  Top 0.305: LED1.7 34.8,83.31 33.02,83.31 v33.02,56.13 | R1.2 v37.08,54.86
  Bottom 0.305: v33.02,56.13 34.29,54.86 v37.08,54.86
N$14
  Bottom 0.305: LED1.1 35.56,59.69 35.56,55.88 48.26,55.88 R5.2
N$15  (via drill 0.61)
  Top 0.305: LED1.9 30.48,80.01 v30.48,60.96
  Bottom 0.305: R6.2 v30.48,60.96
N$16
  Top 0.305: LED1.10 27.94,80.01 27.94,59.69 32.51,55.12 36.07,55.12 36.07,56.39 R7.2
N$17
  Top 0.305: R8.1 IC2.13
N$18
  Top 0.305: R9.1 IC2.12
N$19
  Top 0.305: R10.1 IC2.11
N$20
  Top 0.305: R11.1 IC2.10
N$21
  Top 0.305: R12.1 IC2.9
N$22
  Top 0.305: R13.1 IC2.15
N$23
  Top 0.305: R14.1 IC2.14
N$24
  Top 0.305: LED2.2 45.72,64.77 45.72,45.21 44.45,43.94 43.18,43.94 43.18,36.32 43.94,35.56 46.99,35.56 R11.2
N$25  (via drill 0.61)
  Top 0.305: v49.53,58.93 48.26,57.66 48.26,45.97 45.72,43.43 45.72,38.1 R10.2
  Bottom 0.305: LED2.4 53.09,62.48 53.09,58.93 v49.53,58.93
N$26  (via drill 0.61)
  Top 0.305: LED2.6 56.13,77.22 56.13,48.26 56.64,47.75 v56.64,39.88
  Bottom 0.305: v56.64,39.88 56.64,35.56 43.18,35.56 R9.2
N$27
  Bottom 0.305: LED2.7 47.5,83.31 26.42,83.31 18.29,75.18 2.79,75.18 2.29,74.68 2.29,35.56 38.1,35.56 R8.2
N$28  (via drill 0.61)
  Top 0.305: v52.07,61.72 55.37,58.42 55.37,48.01 55.88,47.5 55.88,41.66 53.85,39.62 v53.85,38.1
  Bottom 0.305: LED2.1 41.91,63.25 47.5,63.25 49.02,61.72 v52.07,61.72 | v53.85,38.1 52.58,36.83 R12.2
N$29  (via drill 0.61)
  Top 0.305: v26.16,42.16 v26.16,75.44
  Bottom 0.305: LED2.9 38.61,75.44 v26.16,75.44 | v26.16,42.16 31.5,36.83 R13.2
N$30  (via drill 0.61)
  Top 0.305: LED2.10 39.12,84.07 27.18,84.07 v27.18,43.18
  Bottom 0.305: v27.18,43.18 32.26,38.1 35.56,38.1 R14.2
N$31  (via drill 0.61)
  Top 0.305: v21.84,61.21 24.89,64.26 24.89,83.06 28.19,86.36 LED9.A
  Bottom 0.305: v21.84,61.21 IC9.14
N$32
  Top 0.305: R15.1 IC3.13
N$33
  Top 0.305: R16.1 IC3.12
N$34
  Top 0.305: R17.1 IC3.11
N$35
  Top 0.305: R18.1 IC3.10
N$36
  Top 0.305: R19.1 IC3.9
N$37
  Top 0.305: R20.1 IC3.15
N$38
  Top 0.305: R21.1 IC3.14
N$39  (via drill 0.61)
  Top 0.305: R18.2 v76.2,61.98
  Bottom 0.305: LED3.2 62.99,64.01 74.17,64.01 v76.2,61.98
N$40  (via drill 0.61)
  Top 0.305: LED3.4 65.53,65.53 v65.53,59.94
  Bottom 0.305: v65.53,59.94 67.06,58.42 72.39,58.42 R17.2
N$41
  Top 0.305: LED3.6 66.55,83.31 62.23,83.31 62.23,60.2 64.77,57.66 64.77,56.64 65.53,55.88 71.12,55.88 R16.2
N$42
  Top 0.305: LED3.7 64.77,80.01 64.77,60.71 64.52,60.45 64.52,59.44 65.53,58.42 68.58,58.42 R15.2
N$43  (via drill 0.61)
  Top 0.305: LED3.1 58.93,65.53 v58.93,57.91
  Bottom 0.305: v58.93,57.91 60.96,55.88 77.47,55.88 R19.2
N$44  (via drill 0.61)
  Top 0.305: LED3.9 59.69,80.01 59.69,59.44 v61.21,57.91
  Bottom 0.305: v61.21,57.91 61.98,57.15 R20.2
N$45  (via drill 0.61)
  Top 0.305: LED3.10 57.15,80.01 v57.15,60.45
  Bottom 0.305: v57.15,60.45 58.67,58.93 64.26,58.93 R21.2
N$46
  Top 0.305: R22.1 IC4.13
N$47
  Top 0.305: R23.1 IC4.12
N$48
  Top 0.305: R24.1 IC4.11
N$49
  Top 0.305: R25.1 IC4.10
N$50
  Top 0.305: R26.1 IC4.9
N$51
  Top 0.305: R27.1 58.42,8.89 58.42,29.21 60.45,31.24 63.5,31.24 IC4.15
N$52
  Top 0.305: R28.1 64.77,27.94 IC4.14
N$53  (via drill 0.61)
  Top 0.305: LED4.2 73.91,65.79 v73.91,62.74 | v78.74,58.93 80.01,57.66 v80.01,38.61
  Bottom 0.305: v73.91,62.74 77.72,58.93 v78.74,58.93 | v80.01,38.61 79.5,38.1 77.47,38.1 R25.2
N$54  (via drill 0.61)
  Top 0.305: LED4.4 81.03,63.75 v81.03,37.59
  Bottom 0.305: v81.03,37.59 81.03,35.56 74.93,35.56 R24.2
N$55  (via drill 0.61)
  Top 0.305: v84.58,43.18 v84.58,82.3
  Bottom 0.305: LED4.6 82.3,82.3 v84.58,82.3 | v84.58,43.18 81.03,39.62 73.91,39.62 R23.2
N$56  (via drill 0.61)
  Top 0.305: v74.93,77.47 74.93,48.26 69.85,43.18 69.85,38.1 R22.2
  Bottom 0.305: v74.93,77.47 LED4.7
N$57  (via drill 0.61)
  Top 0.305: v82.3,57.4 82.3,37.08 81.79,36.58 78.74,36.58 R26.2
  Bottom 0.305: LED4.1 73.15,68.07 74.17,68.07 74.93,67.31 74.93,64.26 75.44,64.26 v82.3,57.4
N$58  (via drill 0.61)
  Top 0.305: LED4.9 67.31,74.93 67.31,64.26 v68.58,62.99 | v41.91,53.85 40.64,52.58 40.64,27.94 45.72,22.86 v45.72,11.43
  Bottom 0.305: v68.58,62.99 68.33,63.25 58.42,63.25 49.02,53.85 v41.91,53.85 | v45.72,11.43 46.99,10.16 61.47,10.16 62.23,9.4 R27.2
N$59
  Top 0.305: LED4.10 73.15,83.31 77.47,83.31 77.47,27.94 72.39,22.86 72.39,14.99 70.87,13.46 70.87,10.92 72.39,9.4 72.39,8.38 71.63,7.62 R28.2
N$60
  Top 0.305: R29.1 IC5.13
N$61
  Top 0.305: R30.1 IC5.12
N$62
  Top 0.305: R31.1 IC5.11
N$63
  Top 0.305: R32.1 IC5.10
N$64
  Top 0.305: R33.1 IC5.9
N$65
  Top 0.305: R34.1 IC5.15
N$66
  Top 0.305: R35.1 IC5.14
N$67
  Bottom 0.305: LED5.2 88.14,68.07 87.12,68.07 86.36,67.31 86.36,55.88 104.14,55.88 R32.2
N$68  (via drill 0.61)
  Top 0.305: v102.62,62.23 102.87,61.98 R31.2
  Bottom 0.305: LED5.4 99.06,62.23 v102.62,62.23
N$69
  Top 0.305: LED5.6 98.3,80.77 98.3,68.07 99.06,67.31 99.06,58.42 R30.2
N$70
  Top 0.305: LED5.7 96.52,80.01 96.52,58.67 97.79,57.4 R29.2
N$71
  Bottom 0.305: LED5.1 95.25,58.42 106.68,58.42 R33.2
N$72
  Top 0.305: LED5.9 91.95,79.5 91.95,67.82 91.44,67.31 91.44,58.42 R34.2
N$73
  Top 0.305: LED5.10 89.66,83.31 93.98,83.31 93.98,58.42 R35.2
N$74
  Top 0.305: R36.1 IC6.13
N$75
  Top 0.305: R37.1 IC6.12
N$76
  Top 0.305: R38.1 IC6.11
N$77
  Top 0.305: R39.1 IC6.10
N$78
  Top 0.305: R40.1 IC6.9
N$79
  Top 0.305: R41.1 IC6.15
N$80
  Top 0.305: R42.1 IC6.14
N$81
  Top 0.305: LED6.2 106.68,62.23 106.68,39.88 109.22,37.34 109.22,36.32 108.46,35.56 105.41,35.56 R39.2
N$82  (via drill 0.61)
  Top 0.305: v95.5,59.69 95.76,59.44 95.76,58.42 96.52,57.66 96.52,48.26 101.6,43.18 101.6,38.35 102.87,37.08 R38.2
  Bottom 0.305: LED6.4 101.6,59.69 v95.5,59.69
N$83  (via drill 0.61)
  Top 0.305: v90.93,72.64 86.36,68.07 86.36,46.48 88.9,43.94 88.9,38.86 92.2,35.56 100.33,35.56 R37.2
  Bottom 0.305: LED6.6 108.46,83.31 92.2,83.31 91.44,82.55 91.44,72.64 v90.93,72.64
N$84  (via drill 0.61)
  Top 0.305: v90.93,71.12 88.9,69.09 88.9,53.34 91.44,50.8 91.44,48.26 96.52,43.18 96.52,38.1 R36.2
  Bottom 0.305: LED6.7 97.79,71.12 v90.93,71.12
N$85
  Top 0.305: LED6.1 101.6,64.77 101.6,45.72 104.14,43.18 104.14,40.64 R40.2
N$86  (via drill 0.61)
  Top 0.305: LED6.9 100.84,79.25 99.06,79.25 99.06,82.55 97.54,84.07 83.57,84.07 v83.57,40.64
  Bottom 0.305: v83.57,40.64 87.38,36.83 R41.2
N$87  (via drill 0.61)
  Top 0.305: LED6.10 102.36,83.31 106.68,83.31 106.68,63.25 107.7,62.23 107.7,59.18 109.22,57.66 v109.22,40.13
  Bottom 0.305: v109.22,40.13 107.19,38.1 96.52,38.1 R42.2
N$88
  Top 0.305: R43.1 IC7.13
N$89
  Top 0.305: R44.1 IC7.12
N$90
  Top 0.305: R45.1 IC7.11
N$91
  Top 0.305: R46.1 IC7.10
N$92
  Top 0.305: R47.1 IC7.9
N$93
  Top 0.305: R48.1 IC7.15
N$94
  Top 0.305: R49.1 IC7.14
N$95
  Bottom 0.305: LED7.2 123.19,58.42 129.54,58.42 R46.2
N$96
  Top 0.305: LED7.4 121.16,65.53 121.16,58.42 121.92,57.66 121.92,56.64 122.68,55.88 128.27,55.88 R45.2
N$97
  Top 0.305: LED7.6 124.46,80.01 124.46,58.42 R44.2
N$98
  Top 0.305: LED7.7 121.92,80.01 121.92,58.67 123.19,57.4 R43.2
N$99
  Bottom 0.305: LED7.1 111,68.07 109.98,68.07 109.22,67.31 109.22,63.25 108.71,63.25 107.7,62.23 107.7,58.42 115.06,58.42 117.6,55.88 132.08,55.88 R47.2
N$100
  Top 0.305: LED7.9 117.6,83.31 119.38,83.31 119.38,58.42 R48.2
N$101
  Top 0.305: LED7.10 116.84,77.47 116.84,56.64 117.6,55.88 120.65,55.88 R49.2
N$102
  Top 0.305: R50.1 IC8.13
N$103
  Top 0.305: R51.1 IC8.12
N$104
  Top 0.305: R52.1 IC8.11
N$105
  Top 0.305: R53.1 IC8.10
N$106
  Top 0.305: R54.1 IC8.9
N$107
  Top 0.305: R55.1 IC8.15
N$108
  Top 0.305: R56.1 IC8.14
N$109  (via drill 0.61)
  Top 0.305: v134.62,59.69 134.62,45.72 132.08,43.18 132.08,38.35 130.81,37.08 R53.2
  Bottom 0.305: v134.62,59.69 LED8.2
N$110
  Top 0.305: LED8.4 135.64,63.75 135.64,40.89 132.08,37.34 132.08,36.32 131.32,35.56 128.27,35.56 R52.2
N$111  (via drill 0.61)
  Top 0.305: LED8.6 137.92,79.25 v137.92,43.94
  Bottom 0.305: v137.92,43.94 132.08,38.1 127,38.1 R51.2
N$112
  Top 0.305: LED8.7 132.08,80.01 132.08,48.26 127,43.18 127,40.64 R50.2
N$113  (via drill 0.61)
  Top 0.305: v136.91,58.42 136.65,58.17 136.65,40.13 R54.2
  Bottom 0.305: LED8.1 133.35,58.42 v136.91,58.42
N$114
  Bottom 0.305: LED8.9 138.94,70.61 138.94,35.56 119.38,35.56 R55.2
N$115
  Top 0.305: LED8.10 129.54,77.47 129.54,55.12 127,52.58 127,48.26 121.92,43.18 121.92,38.1 R56.2
N$116  (via drill 0.61)
  Top 0.305: IC9.15 10.16,52.07 v10.16,77.72
  Bottom 0.305: v10.16,77.72 17.53,85.09 57.15,85.09 LED11.A
N$117
  Bottom 0.305: IC9.1 5.08,45.47 4.32,45.47 3.05,46.74 3.05,74.42 49.02,74.42 60.96,86.36 LED12.A
N$118
  Bottom 0.305: IC9.6 13.46,46.23 4.57,46.23 3.81,46.99 3.81,73.66 73.66,73.66 80.01,80.01 80.01,86.36 LED13.A
N$119  (via drill 0.61)
  Top 0.305: IC9.7 16.51,45.72 v16.51,60.71
  Bottom 0.305: v16.51,60.71 11.18,66.04 11.18,71.88 75.69,71.88 90.17,86.36 LED14.A
N$120
  Top 0.305: IC9.4 11.43,43.18 11.43,65.79 11.18,66.04 11.18,88.9 12.45,90.17 102.87,90.17 102.87,87.63 LED15.A
N$121
  Bottom 0.305: LED16.K 123.19,91.44 R58.1
N$123
  Bottom 0.305: LED16.A 121.92,87.63 Q1.E
S
  Bottom 0.305: X1.25 72.39,8.89 72.39,5.84 73.15,5.08 143.51,5.08 143.51,85.6 Q1.B
T10  (via drill 0.61)
  Top 0.305: IC2.7 48.26,22.86 48.26,44.96 50.8,47.5 v50.8,53.09 | v93.73,53.34 93.98,53.09 93.98,48.26 99.06,43.18 99.06,39.88 101.6,37.34 101.6,11.43 X1.3
  Bottom 0.305: v50.8,53.09 51.05,53.34 v93.73,53.34
T11
  Bottom 0.305: IC2.1 39.37,13.97 79.76,13.97 82.04,11.68 95.5,11.68 97.79,9.4 97.79,6.35 X1.4
T12  (via drill 0.61)
  Top 0.305: v81.03,15.75 82.8,13.97 v82.8,10.67
  Bottom 0.305: IC2.2 40.13,15.75 v81.03,15.75 | v82.8,10.67 83.31,10.16 95.25,10.16 X1.5
T13  (via drill 0.61)
  Top 0.305: IC2.6 44.2,21.34 v44.2,5.08 | X1.6 v94.23,4.06
  Bottom 0.305: v44.2,5.08 45.21,4.06 v94.23,4.06
T100  (via drill 0.61)
  Top 0.305: v54.86,39.12 55.88,38.1 v55.88,11.94
  Bottom 0.305: IC1.7 49.78,39.12 v54.86,39.12 | v55.88,11.94 56.9,10.92 66.55,10.92 67.31,10.16 81.79,10.16 82.55,9.4 82.55,7.62 92.71,7.62 X1.7
T101  (via drill 0.61)
  Top 0.305: v87.38,33.02 88.9,31.5 88.9,27.94 93.98,22.86 93.98,10.67 95.25,9.4 95.25,7.62 X1.8
  Bottom 0.305: IC1.1 34.8,38.86 39.12,38.86 40.64,37.34 40.64,33.02 v87.38,33.02
TA_CLK  (via drill 0.61)
  Top 0.305: v39.37,11.43 38.1,12.7 38.1,43.18 33.02,48.26 v33.02,54.1
  Bottom 0.305: X1.32 62.23,5.08 45.72,5.08 v39.37,11.43 | v33.02,54.1 19.81,67.31 S5.3
TA_CLR  (via drill 0.61)
  Top 0.305: X1.31 62.23,10.16 v62.23,25.4 | v31.5,25.4 21.59,35.31 21.59,59.94 19.3,62.23 19.3,75.95 S6.3
  Bottom 0.305: v31.5,25.4 v62.23,25.4
TA_J  (via drill 0.61)
  Top 0.305: X1.29 66.29,9.14 66.29,19.3 67.31,20.32 v67.31,34.04 | v108.46,34.54 114.3,40.39 S3.3
  Bottom 0.305: v67.31,34.04 67.82,34.54 v108.46,34.54
TA_M  (via drill 0.61)
  Top 0.305: X1.28 67.31,7.62 v67.31,11.68 | v57.4,11.94 57.66,12.19 57.66,48.77 64.01,55.12 72.39,55.12 S2.3
  Bottom 0.305: v67.31,11.68 67.06,11.94 v57.4,11.94
TA_T  (via drill 0.61)
  Top 0.305: X1.27 69.85,10.16 69.85,33.02 62.23,40.64 62.23,43.18 v59.69,45.72 | v44.7,45.72 43.18,47.24 S1.3
  Bottom 0.305: v44.7,45.72 v59.69,45.72
TA_W
  Top 0.305: X1.30 64.77,5.08 52.83,5.08 52.83,59.44 48.26,64.01 48.26,82.55 43.18,87.63 S4.3
W0  (via drill 0.61)
  Top 0.305: IC9.10 20.07,49.28 v20.07,44.2 | v12.95,36.58 13.21,36.32 13.21,29.72 41.4,1.52 76.2,1.52 X1.22
  Bottom 0.305: v20.07,44.2 19.05,43.18 19.05,36.58 v12.95,36.58
W1  (via drill 0.61)
  Top 0.305: IC9.13 13.97,48.26 13.97,30.48 v31.5,12.95 | v71.88,12.95 73.66,11.18 X1.23
  Bottom 0.305: v71.88,12.95 v31.5,12.95
W2
  Top 0.305: IC9.12 15.75,49.02 15.75,43.94 16.51,43.18 16.51,29.46 43.69,2.29 73.66,2.29 X1.24

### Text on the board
Top: Datumsanzeige 2000-2099
Bottom: Datumsanzeige 2000-2099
